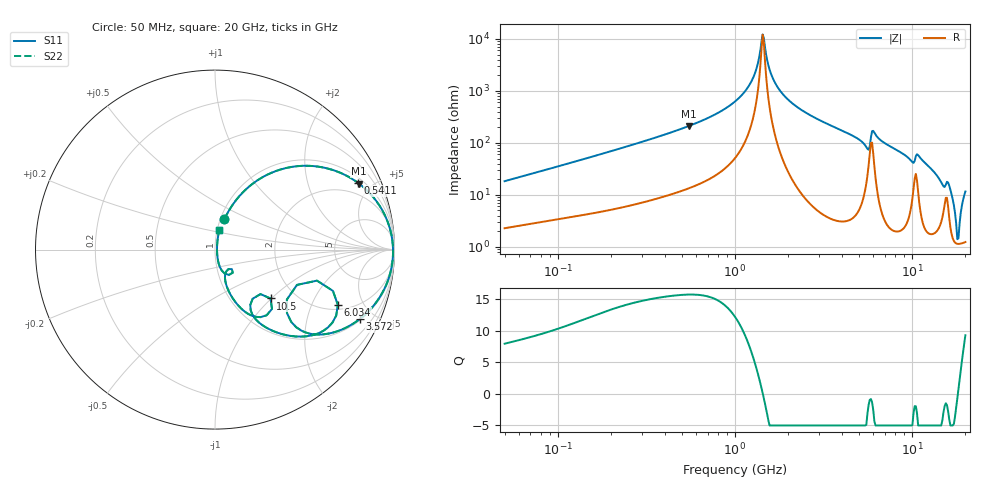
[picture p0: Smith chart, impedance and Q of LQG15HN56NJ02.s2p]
!Murata Part Number: LQG15HN56NJ02
!These Parameters are Measured in Series Mode Connection
!  o--[Z]--o
!Port1  Port2
!  o-------o
!Freq. Start=50[MHz] Stop=20[GHz], 401[Steps]
# Hz S RI R 50
!Freq.(Hz) S11(Real) S11(Imag) S21(Real) S21(Imag) S12(Real) S12(Imag) S22(Real) S22(Imag)
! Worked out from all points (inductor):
!   401 points, 50 MHz to 20 GHz, reference 50 ohm
!   read as one part in series: L = 56.9 nH near 51.52 MHz
!   highest Q = 15.8 at 549.3 MHz (marker M1), where L = 61.1 nH
!   self-resonance near 1.433 GHz
!   S11 on the Smith chart (normalised r, x): 50 MHz: 1.05, +0.36; 541.1 MHz: 1.26, +4.14; 3.572 GHz: 1.07, -4.14; 6.034 GHz: 2.25, -3.17; 10.5 GHz: 1.51, -0.99; 20 GHz: 1.02, +0.23
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5e7  0.0522 0.1684  0.9478 -0.1684  0.9478 -0.1684  0.0522 0.1684
1.364002e8  0.2041 0.3625  0.7959 -0.3625  0.7959 -0.3625  0.2041 0.3625
3.721004e8  0.6303 0.4511  0.3697 -0.4511  0.3697 -0.4511  0.6303 0.4511
5.411141e8  0.7966 0.3721  0.2034 -0.3721  0.2034 -0.3721  0.7966 0.3721
5.492803e8  0.8024 0.3678  0.1976 -0.3678  0.1976 -0.3678  0.8024 0.3678
1e9  0.9633 0.1517  0.0367 -0.1517  0.0367 -0.1517  0.9633 0.1517
1.251922e9  0.987 0.0585  0.013 -0.0585  0.013 -0.0585  0.987 0.0585
1.432596e9  0.9919 0.00119  0.00805 -0.00119  0.00805 -0.00119  0.9919 0.00119
1.590961e9  0.9909 -0.0439  0.00912 0.0439  0.00912 0.0439  0.9909 -0.0439
1.766834e9  0.9854 -0.0894  0.0146 0.0894  0.0146 0.0894  0.9854 -0.0894
2.728004e9  0.909 -0.2783  0.091 0.2783  0.091 0.2783  0.909 -0.2783
3.572216e9  0.8068 -0.3868  0.1932 0.3868  0.1932 0.3868  0.8068 -0.3868
5.041459e9  0.5655 -0.4732  0.4345 0.4732  0.4345 0.4732  0.5655 -0.4732
5.598765e9  0.4008 -0.3532  0.5992 0.3532  0.5992 0.3532  0.4008 -0.3532
6.034176e9  0.6843 -0.3074  0.3157 0.3074  0.3157 0.3074  0.6843 -0.3074
7.442007e9  0.4351 -0.4827  0.5649 0.4827  0.5649 0.4827  0.4351 -0.4827
9.745021e9  0.2074 -0.3603  0.7926 0.3603  0.7926 0.3603  0.2074 -0.3603
1.050288e10  0.3095 -0.2724  0.6905 0.2724  0.6905 0.2724  0.3095 -0.2724
1.621653e10  0.0529 -0.1325  0.9471 0.1325  0.9471 0.1325  0.0529 -0.1325
1.800918e10  0.0114 -0.00795  0.9886 0.00795  0.9886 0.00795  0.0114 -0.00795
1.855685e10  0.012 0.0259  0.988 -0.0259  0.988 -0.0259  0.012 0.0259
2e10  0.0249 0.1111  0.9751 -0.1111  0.9751 -0.1111  0.0249 0.1111
